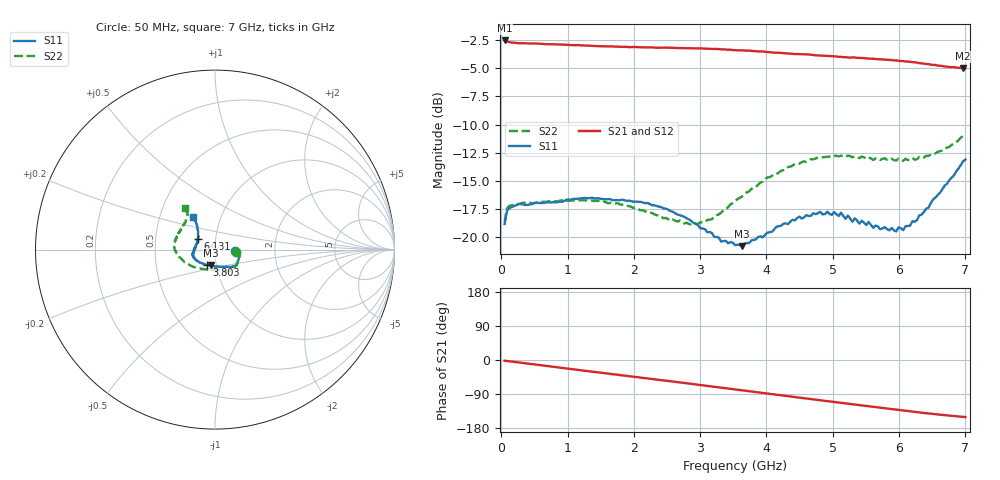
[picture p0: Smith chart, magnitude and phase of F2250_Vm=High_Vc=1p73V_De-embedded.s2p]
! Integrated Device Technology
! Corporate Headquarters
! 6024 Silver Creek Valley Road
! San Jose, CA 95138  USA
! Phone:  1-408-284-8200
! Toll Free:  1-800-223-1366
! Webpage:  http://www.idt.com/
! Timing and RF Division
! 515 Groton Road, Suite 102
! Westford, MA 01886-6024
! Device:  F2250
! Description: Voltage Variable RF Attenuator
! Frequency:  50.0 -  6000.00 MHz
! Package:  3x3 mm Thin QFN Plastic Package: 16 pin
! Ports:  2 RF, 3 DC
!  Pin  1  = GND
!  Pin  2  = NC
!  Pin  3  = RF1  = Port 1
!  Pin  4  = NC
!  Pin  5  = GND
!  Pin  6  = GND
!  Pin  7  = GND
!  Pin  8  = GND
!  Pin  9  = NC
!  Pin 10  = RF2  = Port 2
!  Pin 11  = NC
!  Pin 12  = GND
!  Pin 13  = GND
!  Pin 14  = VCNTRL
!  Pin 15  = VDD
!  Pin 16  = VMODE
! Vcntrl:  1.730 Volts
! Vmode:  +3.300 Volts
! Vdd:  +3.30  Volts
! Current:  1.325 mA
! Data:  The device was measured on a the F2250 evaluation board which has
!  individual transmission lines to the RF pins.  Data was collected
!  using a calibrated network analyzer.  The evaluation board was
!  de-embedded using a TRL calibration technique.
!  The reference plane is the edge of the package pin.
! Misc:  SN 10
!  Action Tracker AT0258
! Date Measured:  2014-11-26
! Date:  2015-10-15  MJV
! Note:
!  Integrated Device Technology supplies this data as a sample of measured
!  data at the package pin for this product.  Your particular data for this
!  product may vary.
!  Data was taken at 25 degrees C.
!  Integrated Device Technology reserves the right to change this data at anytime.
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# GHz S dB R 50
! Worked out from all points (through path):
!   201 points, 50 MHz to 7 GHz, reference 50 ohm
!   highest |S21| = -2.51 dB at 50 MHz (marker M1); lowest = -5.0 dB at 6.965 GHz (marker M2)
!   group delay of S21, straight-line fit = 60.5 ps
!   lowest |S11| = -20.8 dB at 3.629 GHz (marker M3), VSWR 1.20, Z = 47.2 - j8.4 ohm
!   |S11| at or under -10 dB: start of sweep to end of sweep
!   |S22| runs from -18.9 to -10.9 dB; largest |S21 - S12| = 0.0035
!   S11 on the Smith chart (normalised r, x): 50 MHz: 1.26, -0.02; 3.803 GHz: 0.90, -0.16; 6.131 GHz: 0.82, +0.10; 7 GHz: 0.73, +0.28
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0.05  -18.86 -4.8  -2.51 -2.0  -2.52 -2.0  -18.65 -5.9
0.08475  -17.70 -4.4  -2.60 -2.6  -2.63 -2.6  -17.49 -5.3
0.2585  -17.09 -9.4  -2.76 -6.4  -2.76 -6.4  -17.08 -12.3
1.2315  -16.56 -34.8  -2.96 -27.8  -2.96 -27.8  -16.74 -47.2
1.75275  -16.73 -41.2  -3.07 -38.8  -3.07 -38.8  -17.01 -59.0
2.37825  -17.31 -44.5  -3.16 -52.2  -3.15 -52.2  -18.07 -72.6
2.969  -18.99 -57.9  -3.21 -65.3  -3.23 -65.3  -18.85 -100.1
3.3165  -20.43 -78.8  -3.31 -73.1  -3.29 -73.2  -17.84 -122.9
3.525  -20.74 -94.4  -3.38 -77.8  -3.36 -77.9  -16.87 -134.7
3.62925  -20.84 -103.5  -3.39 -80.2  -3.38 -80.3  -16.43 -140.0
3.803  -20.28 -116.7  -3.45 -84.1  -3.45 -84.1  -15.62 -148.0
4.4285  -18.54 -149.1  -3.72 -97.9  -3.70 -97.9  -13.50 -171.7
4.7065  -17.90 -159.3  -3.81 -104.0  -3.81 -104.0  -13.11 -178.6
5.1235  -17.85 -170.0  -3.97 -113.0  -3.95 -113.1  -12.79 171.3
5.29725  -18.67 -174.9  -4.02 -116.7  -4.01 -116.8  -12.92 167.7
5.332  -18.35 -176.8  -4.03 -117.6  -4.03 -117.6  -12.84 166.7
5.4015  -18.83 -177.9  -4.07 -119.0  -4.04 -119.1  -12.99 164.7
5.85325  -19.43 163.9  -4.25 -128.7  -4.22 -128.8  -13.15 152.7
6.13125  -19.04 148.8  -4.39 -134.6  -4.39 -134.7  -13.17 145.0
6.444  -17.39 133.7  -4.61 -141.2  -4.64 -141.3  -12.80 134.8
6.96525  -13.28 124.3  -4.99 -150.1  -4.98 -150.2  -11.03 126.1
7  -13.12 124.0  -4.99 -150.6  -5.01 -150.7  -10.90 125.4
